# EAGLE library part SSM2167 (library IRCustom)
SSM2167 Microphone conditioner chip
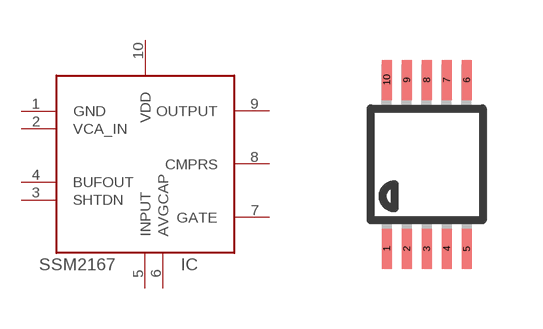
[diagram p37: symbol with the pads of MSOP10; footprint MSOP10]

Designator prefix IC

## SSM2167  [MSOP10]
1  GND  pwr
2  VCA_IN  in
3  SHTDN  in
4  BUFOUT  out
5  INPUT  in
6  AVGCAP  pas
7  GATE  pas
8  CMPRS  pas
9  OUTPUT  out
10  VDD  pwr

## Footprint MSOP10 (pad centres in mm)
10-Lead Mini Small Outline Package [MSOP]
smd 0.25 x 1: 1 -1,-2.113; 2 -0.5,-2.113; 3 0,-2.113; 4 0.5,-2.113; 5 1,-2.113; 6 1,2.113; 7 0.5,2.113; 8 0,2.113; 9 -0.5,2.113; 10 -1,2.113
